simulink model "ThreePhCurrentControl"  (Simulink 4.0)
settings: Solver=ode23  StartTime=-eps  StopTime=0.2  FixedStep=0.000001  RelTol=1e-3
undefined symbols (not defined in the file or in its folder): di, Element, L, R, sfunxy, Symmetrized, Ts, Udc, Upp, Warning
libraries: simulink3 x1

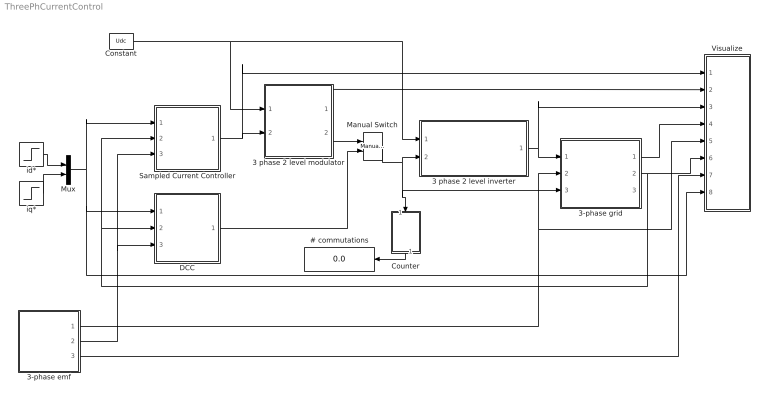
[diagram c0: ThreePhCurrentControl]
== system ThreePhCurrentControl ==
  # commutations : Display
  3 phase 2 level inverter : Subsystem  SimViewingDevice=off
  3 phase 2 level modulator : Subsystem  SimViewingDevice=off  mask{type=Symmetrized, Random=Fixed frequency, Ts=Ts}
      mask prompts: type "Sinus, Symmetrized or Minimum switch modulation"; Random "Fixed or random modulation?"; Ts "Sampling interval"
      mask help: Carrier Wave modulator that uses either fixed frequency modulation or random modulation. The fixed frequency modulation uses 1/(2Ts) as modulation frequency. The random modulation selects the modulatio frequency by random every sampling instant. The selection uses either 1/Ts, 1/(2Ts) or 1/(3Ts) as carrier wave frequency.
  3-phase emf : Subsystem  SimViewingDevice=off  mask{Upp=Upp, freq=50, Tc=0.1e-3}
      mask prompts: Upp "U_phase_to_phase [RMS]"; freq "Frequency"; Tc "Sampling time"
  3-phase grid : Subsystem  SimViewingDevice=off  mask{L=L, R=R}
      mask prompts: L "Inductance [H]"; R "Resistance [ohm]"
  Constant : Constant  Value=Udc
  Counter : Subsystem  Orientation=down  SimViewingDevice=off
  DCC : Subsystem  SimViewingDevice=off
  Manual Switch : simulink3/Nonlinear/Manual Switch  sw=0  action=0
  Mux : Mux  Inputs=2
  Sampled Current Controller : Subsystem  SimViewingDevice=off  mask{R=R, L=L, Kp=(L/Ts+R/2), Ti=L/R+Ts/2, Ts=Ts, Umax=Udc, Umin=-Udc, SlowFast=Slow Computer}
      mask prompts: R "Load resistance"; L "Load inductance"; Kp "Controller gain"; Ti "Integral Time Constant"; Ts "Sampling time [s]"; Umax "Max output signal"; Umin "Min output signal"; SlowFast "Controller type"
  Visualize : Subsystem  SimViewingDevice=off
  id* : Step  Time=0.0105  Before=0  After=-10  SampleTime=0
  iq* : Step  Time=0.0055  Before=0  After=10  SampleTime=0
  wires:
  3 phase 2 level inverter/1(va,b,c) -> 3-phase grid/1(va,b,c), Visualize/3(v)
  Sampled Current Controller/1(u*) -> 3 phase 2 level modulator/2(uabc*), Visualize/1(u*)
  Constant/1 -> 3 phase 2 level inverter/1(Udc), 3 phase 2 level modulator/1(Udc)
  Counter/1(#) -> # commutations/1
  3 phase 2 level modulator/2(sa,b,c) -> Manual Switch/1
  Manual Switch/1 -> 3 phase 2 level inverter/2(sa,b,c), Counter/1(sa,b,c), 3-phase grid/3(s)
  DCC/1(sa,b,c) -> Manual Switch/2
  3 phase 2 level modulator/1(mod) -> Visualize/2(mod)
  3-phase emf/1(e_line) -> 3-phase grid/2(e_line), Visualize/5(e)
  3-phase grid/1(u_ab) -> Visualize/4("u ")
  3-phase grid/2(i_ab) -> Visualize/6(i), DCC/2(Act_ab), Sampled Current Controller/2(Act_ab)
  3-phase emf/3(Theta_line) -> Visualize/7(theta)
  3-phase emf/2(Psi_line) -> DCC/3(psi), Sampled Current Controller/3(psi)
  id*/1 -> Mux/1
  iq*/1 -> Mux/2
  Mux/1 -> Sampled Current Controller/1(Ref_dq), DCC/1(Ref_dq), Visualize/8(i*dq)

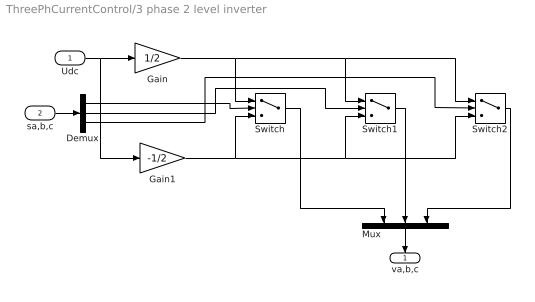
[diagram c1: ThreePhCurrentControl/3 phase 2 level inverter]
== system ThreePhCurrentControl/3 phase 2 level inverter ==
  Udc : Inport  Port=1  PortDimensions=-1  SampleTime=-1  DataType=auto
  sa,b,c : Inport  Port=2  PortDimensions=-1  SampleTime=-1  DataType=auto
  Demux : Demux  Outputs=3  BusSelectionMode=off
  Gain : Gain  Gain=1/2  Multiplication=Element-wise(K.*u)  SaturateOnIntegerOverflow=on
  Gain1 : Gain  Gain=-1/2  Multiplication=Element-wise(K.*u)  SaturateOnIntegerOverflow=on
  Mux : Mux  Orientation=down  Inputs=3
  Switch : Switch  Threshold=0
  Switch1 : Switch  Threshold=0
  Switch2 : Switch  Threshold=0
  va,b,c : Outport  Orientation=down  Port=1  InitialOutput=0
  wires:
  Gain/1 -> Switch/1, Switch1/1, Switch2/1
  Gain1/1 -> Switch/3, Switch1/3, Switch2/3
  Udc/1 -> Gain1/1, Gain/1
  sa,b,c/1 -> Demux/1
  Demux/1 -> Switch/2
  Demux/2 -> Switch1/2
  Demux/3 -> Switch2/2
  Switch/1 -> Mux/1
  Switch1/1 -> Mux/2
  Switch2/1 -> Mux/3
  Mux/1 -> va,b,c/1

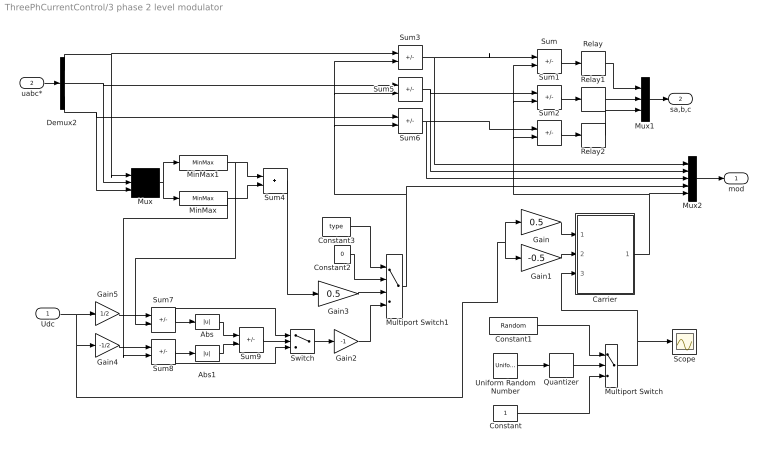
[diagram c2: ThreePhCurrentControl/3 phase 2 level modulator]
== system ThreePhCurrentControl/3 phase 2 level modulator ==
  Udc : Inport  Port=1  PortDimensions=-1  SampleTime=-1  DataType=auto
  uabc* : Inport  Port=2  PortDimensions=-1  SampleTime=-1  DataType=auto
  Abs : Abs  SaturateOnIntegerOverflow=on
  Abs1 : Abs  SaturateOnIntegerOverflow=on
  Carrier : Subsystem  SimViewingDevice=off
  Constant : Constant  Value=1
  Constant1 : Constant  Value=Random
  Constant2 : Constant  Value=0
  Constant3 : Constant  Value=type
  Demux2 : Demux  Outputs=3  BusSelectionMode=off
  Gain : Gain  Gain=0.5  Multiplication=Element-wise(K.*u)  SaturateOnIntegerOverflow=on
  Gain1 : Gain  Gain=-0.5  Multiplication=Element-wise(K.*u)  SaturateOnIntegerOverflow=on
  Gain2 : Gain  Gain=-1  Multiplication=Element-wise(K.*u)  SaturateOnIntegerOverflow=on
  Gain3 : Gain  Gain=0.5  Multiplication=Element-wise(K.*u)  SaturateOnIntegerOverflow=on
  Gain4 : Gain  Gain=-1/2  Multiplication=Element-wise(K.*u)  SaturateOnIntegerOverflow=on
  Gain5 : Gain  Gain=1/2  Multiplication=Element-wise(K.*u)  SaturateOnIntegerOverflow=on
  MinMax : MinMax  Function=min  Inputs=1
  MinMax1 : MinMax  Function=max  Inputs=1
  Multiport Switch : MultiPortSwitch  Inputs=2
  Multiport Switch1 : MultiPortSwitch  Inputs=3
  Mux : Mux  Inputs=3
  Mux1 : Mux  Inputs=3
  Mux2 : Mux  Inputs=5
  Quantizer : Quantizer  QuantizationInterval=1  LinearizeAsGain=on
  Relay : Relay  OnSwitchValue=eps  OffSwitchValue=eps  OnOutputValue=1  OffOutputValue=-1
  Relay1 : Relay  OnSwitchValue=eps  OffSwitchValue=eps  OnOutputValue=1  OffOutputValue=-1
  Relay2 : Relay  OnSwitchValue=eps  OffSwitchValue=eps  OnOutputValue=1  OffOutputValue=-1
  Scope : Scope
  Sum{,1..3,5..8} (8 alike) : Sum  Inputs=+-  SaturateOnIntegerOverflow=on
  Sum4 : Sum  Inputs=++  SaturateOnIntegerOverflow=on
  Sum9 : Sum  Inputs=-+  SaturateOnIntegerOverflow=on
  Switch : Switch  Threshold=0
  Uniform Random Number : UniformRandomNumber  Minimum=1  Maximum=3  Seed=0.9874  SampleTime=Ts
  mod : Outport  Port=1  InitialOutput=0
  sa,b,c : Outport  Port=2  InitialOutput=0
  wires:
  Carrier/1(um) -> Sum2/2, Sum1/2, Sum/2, Mux2/5
  Gain1/1 -> Carrier/2(Umin)
  Gain/1 -> Carrier/1(Umax)
  Sum/1 -> Relay/1
  Relay1/1 -> Mux1/2
  Sum1/1 -> Relay1/1
  Relay2/1 -> Mux1/3
  Sum2/1 -> Relay2/1
  Quantizer/1 -> Multiport Switch/2
  Uniform Random Number/1 -> Quantizer/1
  Constant/1 -> Multiport Switch/3
  Multiport Switch/1 -> Carrier/3(x), Scope/1
  Constant1/1 -> Multiport Switch/1
  Sum3/1 -> Mux2/1, Sum/1
  Sum5/1 -> Mux2/2, Sum1/1
  Sum6/1 -> Mux2/3, Sum2/1
  Demux2/1 -> Sum3/1, Mux/1
  Demux2/2 -> Sum5/1, Mux/2
  Demux2/3 -> Sum6/1, Mux/3
  Mux/1 -> MinMax1/1, MinMax/1
  MinMax1/1 -> Sum4/1, Sum7/2
  MinMax/1 -> Sum4/2, Sum8/2
  Udc/1 -> Gain5/1, Gain4/1, Gain1/1, Gain/1
  Gain4/1 -> Sum8/1
  Sum7/1 -> Abs/1, Switch/1
  Sum8/1 -> Abs1/1, Switch/3
  Abs/1 -> Sum9/1
  Abs1/1 -> Sum9/2
  Sum9/1 -> Switch/2
  Sum4/1 -> Gain3/1
  Switch/1 -> Gain2/1
  Constant3/1 -> Multiport Switch1/1
  Constant2/1 -> Multiport Switch1/2
  Gain3/1 -> Multiport Switch1/3
  Gain2/1 -> Multiport Switch1/4
  Multiport Switch1/1 -> Sum5/2, Sum3/2, Sum6/2, Mux2/4
  Gain5/1 -> Sum7/1
  uabc*/1 -> Demux2/1
  Relay/1 -> Mux1/1
  Mux1/1 -> sa,b,c/1
  Mux2/1 -> mod/1

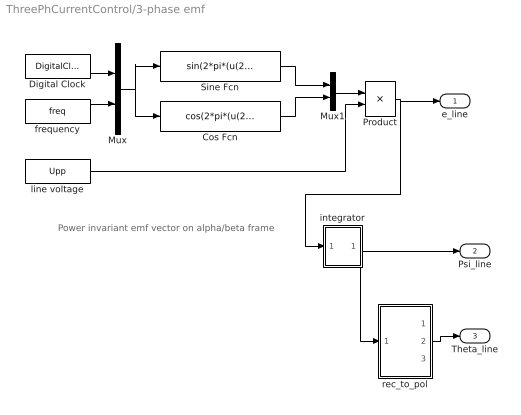
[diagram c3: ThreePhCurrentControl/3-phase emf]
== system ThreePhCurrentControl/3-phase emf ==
  note: Power invariant emf vector on alpha/beta frame
  Cos Fcn : Fcn  Expr=cos(2*pi*(u(2))*u(1))
  Digital Clock : DigitalClock  SampleTime=Tc
  Mux : Mux  Inputs=2
  Mux1 : Mux  Inputs=2
  Product : Product  Inputs=2  Multiplication=Element-wise(.*)  SaturateOnIntegerOverflow=on
  Sine Fcn : Fcn  Expr=sin(2*pi*(u(2))*u(1)-pi)
  frequency : Constant  Value=freq
  integrator : Subsystem  SimViewingDevice=off
  line voltage : Constant  Value=Upp
  rec_to_pol : Subsystem  SimViewingDevice=off
  e_line : Outport  Port=1  InitialOutput=0
  Psi_line : Outport  Port=2  InitialOutput=0
  Theta_line : Outport  Port=3  InitialOutput=0
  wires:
  Product/1 -> e_line/1, integrator/1(In1)
  Mux1/1 -> Product/1
  Cos Fcn/1 -> Mux1/2
  Sine Fcn/1 -> Mux1/1
  Mux/1 -> Cos Fcn/1, Sine Fcn/1
  Digital Clock/1 -> Mux/1
  frequency/1 -> Mux/2
  line voltage/1 -> Product/2
  integrator/1(Out1) -> Psi_line/1, rec_to_pol/1(rect)
  rec_to_pol/2(angle) -> Theta_line/1

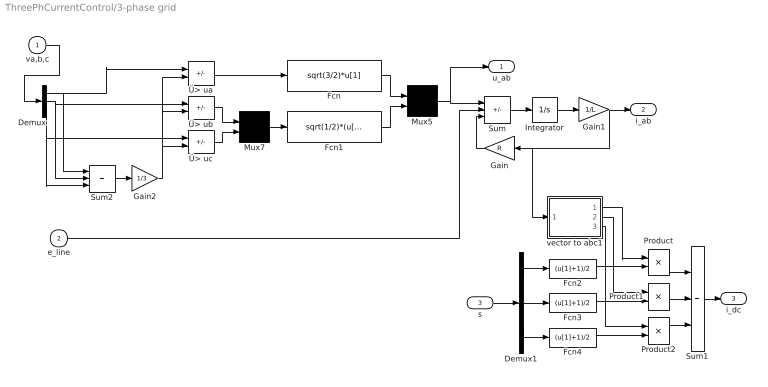
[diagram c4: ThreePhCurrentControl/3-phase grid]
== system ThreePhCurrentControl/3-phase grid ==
  va,b,c : Inport  Port=1  PortDimensions=-1  SampleTime=-1  DataType=auto
  e_line : Inport  Port=2  PortDimensions=-1  SampleTime=-1  DataType=auto
  s : Inport  Port=3  PortDimensions=-1  SampleTime=-1  DataType=auto
  Demux : Demux  Outputs=3  BusSelectionMode=off
  Demux1 : Demux  Outputs=3  BusSelectionMode=off
  Fcn : Fcn  Expr=sqrt(3/2)*u[1]
  Fcn1 : Fcn  Expr=sqrt(1/2)*(u[1]-u[2])
  Fcn2 : Fcn  Expr=(u[1]+1)/2
  Fcn3 : Fcn  Expr=(u[1]+1)/2
  Fcn4 : Fcn  Expr=(u[1]+1)/2
  Gain : Gain  Orientation=left  Gain=R  Multiplication=Element-wise(K.*u)  SaturateOnIntegerOverflow=on
  Gain1 : Gain  Gain=1/L  Multiplication=Element-wise(K.*u)  SaturateOnIntegerOverflow=on
  Gain2 : Gain  Gain=1/3  Multiplication=Element-wise(K.*u)  SaturateOnIntegerOverflow=on
  Integrator : Integrator  ExternalReset=none  InitialConditionSource=internal  InitialCondition=0  LimitOutput=off  UpperSaturationLimit=inf  LowerSaturationLimit=-inf  ShowSaturationPort=off  ShowStatePort=off  AbsoluteTolerance=auto
  Mux5 : Mux  Inputs=2
  Mux7 : Mux  Inputs=2
  Product : Product  Inputs=2  Multiplication=Element-wise(.*)  SaturateOnIntegerOverflow=on
  Product1 : Product  Inputs=2  Multiplication=Element-wise(.*)  SaturateOnIntegerOverflow=on
  Product2 : Product  Inputs=2  Multiplication=Element-wise(.*)  SaturateOnIntegerOverflow=on
  Sum : Sum  Inputs=+--  SaturateOnIntegerOverflow=on
  Sum1 : Sum  Inputs=+++  SaturateOnIntegerOverflow=on
  Sum2 : Sum  Inputs=+++  SaturateOnIntegerOverflow=on
  vector to abc1 : Subsystem  SimViewingDevice=off
  Ü> ua : Sum  Inputs=+-  SaturateOnIntegerOverflow=on
  Ü> ub : Sum  Inputs=+-  SaturateOnIntegerOverflow=on
  Ü> uc : Sum  Inputs=+-  SaturateOnIntegerOverflow=on
  u_ab : Outport  Port=1  InitialOutput=0
  i_ab : Outport  Port=2  InitialOutput=0
  i_dc : Outport  Port=3
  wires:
  Gain1/1 -> i_ab/1, Gain/1, vector to abc1/1(vect)
  Integrator/1 -> Gain1/1
  Gain/1 -> Sum/3
  Sum/1 -> Integrator/1
  Fcn1/1 -> Mux5/2
  Fcn/1 -> Mux5/1
  Mux5/1 -> Sum/1, u_ab/1
  Mux7/1 -> Fcn1/1
  Ü> uc/1 -> Mux7/2
  Ü> ub/1 -> Mux7/1
  Ü> ua/1 -> Fcn/1
  Gain2/1 -> Ü> uc/2, Ü> ub/2, Ü> ua/2
  Demux/2 -> Ü> ub/1, Sum2/2
  Sum2/1 -> Gain2/1
  Demux/3 -> Ü> uc/1, Sum2/3
  Demux/1 -> Ü> ua/1, Sum2/1
  va,b,c/1 -> Demux/1
  Demux1/2 -> Fcn3/1
  Demux1/1 -> Fcn2/1
  Demux1/3 -> Fcn4/1
  s/1 -> Demux1/1
  Sum1/1 -> i_dc/1
  Product2/1 -> Sum1/3
  Product1/1 -> Sum1/2
  Product/1 -> Sum1/1
  vector to abc1/1(a) -> Product/1
  vector to abc1/2(b) -> Product1/1
  vector to abc1/3(c) -> Product2/1
  Fcn4/1 -> Product2/2
  Fcn3/1 -> Product1/2
  Fcn2/1 -> Product/2
  e_line/1 -> Sum/2

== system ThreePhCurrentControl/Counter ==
  sa,b,c : Inport  Port=1  PortDimensions=-1  SampleTime=-1  DataType=auto
  Demux : Demux  Outputs=3  BusSelectionMode=off
  Subsystem : Subsystem  TreatAsAtomicUnit=on  SimViewingDevice=off
  Subsystem1 : Subsystem  TreatAsAtomicUnit=on  SimViewingDevice=off
  Subsystem2 : Subsystem  TreatAsAtomicUnit=on  SimViewingDevice=off
  Sum : Sum  Inputs=+++  SaturateOnIntegerOverflow=on
  # : Outport  Port=1
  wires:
  Sum/1 -> #/1
  Subsystem/1(Out1) -> Sum/2
  Subsystem2/1(Out1) -> Sum/1
  Subsystem1/1(Out1) -> Sum/3
  sa,b,c/1 -> Demux/1
  Demux/2 -> Subsystem/Trigger
  Demux/3 -> Subsystem1/Trigger
  Demux/1 -> Subsystem2/Trigger

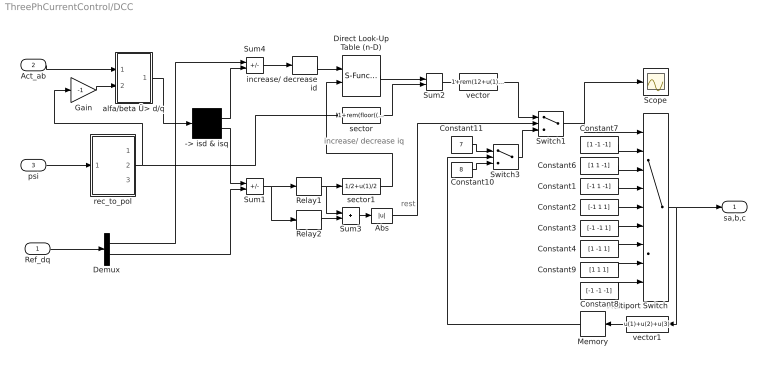
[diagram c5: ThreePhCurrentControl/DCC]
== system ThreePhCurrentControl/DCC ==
  note: increase/ decrease iq
  note: rest
  Ref_dq : Inport  Port=1  PortDimensions=-1  SampleTime=-1  DataType=auto
  Act_ab : Inport  Port=2  PortDimensions=-1  SampleTime=-1  DataType=auto
  psi : Inport  Port=3  PortDimensions=-1  SampleTime=-1  DataType=auto
  -> isd & isq : Demux  Outputs=2  BusSelectionMode=off
  Abs : Abs  SaturateOnIntegerOverflow=on
  Constant1 : Constant  Value=[-1 1 -1]
  Constant10 : Constant  Value=8
  Constant11 : Constant  Value=7
  Constant2 : Constant  Value=[-1 1 1]
  Constant3 : Constant  Value=[-1 -1 1]
  Constant4 : Constant  Value=[1 -1 1]
  Constant6 : Constant  Value=[1 1 -1]
  Constant7 : Constant  Value=[1 -1 -1]
  Constant8 : Constant  Value=[-1 -1 -1]
  Constant9 : Constant  Value=[1 1 1]
  Demux : Demux  Outputs=2  BusSelectionMode=off
  Direct Look-Up Table (n-D) : S-Function  FunctionName=sfun_nddirectlook  Parameters=numInputs,mxTable,clipFlag,tabIsInput,numTDims  PortCounts=[]  SFunctionModules=''  mask(LookupNDDirect){maskTabDims=2, explicitNumDims=1, outDims=Element, tabIsInput=off, mxTable=[4 2;5 1], clipFlag=Warning}
      mask prompts: maskTabDims "Number of table dimensions:"; explicitNumDims "Explicit number of table dimensions:"; outDims "Inputs select this object from table:"; tabIsInput "Make table an input"; mxTable "Table data:"; clipFlag "Action for out of range input:"
      mask help: Table member selection. Inputs are zero-based indices into the table, e.g., an input of 3 returns the fourth element in that dimension. Block can also be used to select a column or 2-D matrix out of the table.
      mask init:
      | if tabIsInput == 1
      |   tWhat = ' T';
      |   yT = 1/(3+maskTabDims-outDims);
      | else
      |   tWhat = ' ';
      |   yT = 0;
      | end
      | if maskTabDims >= 5
      |   numTDims = explicitNumDims;
      | else
      |   numTDims = maskTabDims;
      | end
      | numInputs =  numTDims - (outDims-1);
      | if strcmp(get_param(bdroot(gcb),'BlockDiagramType'),'library')
      |   dimsChar = 'n';
      | else
      |   dimsChar = sprintf('%d',numTDims);
      | end
      | [x,y] = nddirectico('plotdata', numTDims, tabIsInput, outDims);
      | xp = x((end-3):end); yp = y((end-3):end);
      | x = x(1:(end-4)); y = y(1:(end-4));
  Gain : Gain  Gain=-1  Multiplication=Element-wise(K.*u)  SaturateOnIntegerOverflow=on
  Memory : Memory  Orientation=left  X0=0  InheritSampleTime=off
  Multiport Switch : MultiPortSwitch  Inputs=8
  Relay1 : Relay  OnSwitchValue=di/2  OffSwitchValue=-di/2  OnOutputValue=1  OffOutputValue=-1
  Relay2 : Relay  OnSwitchValue=1.3*di/2  OffSwitchValue=-1.3*di/2  OnOutputValue=1  OffOutputValue=-1
  Scope : Scope
  Sum1 : Sum  Inputs=-+  SaturateOnIntegerOverflow=on
  Sum2 : Sum  Inputs=++  SaturateOnIntegerOverflow=on
  Sum3 : Sum  Inputs=++  SaturateOnIntegerOverflow=on
  Sum4 : Sum  Inputs=+-  SaturateOnIntegerOverflow=on
  Switch1 : Switch  Threshold=1
  Switch3 : Switch  Threshold=1
  alfa/beta Ü> d/q : Subsystem  SimViewingDevice=off
  increase/ decrease id : Relay  OnSwitchValue=di/2  OffSwitchValue=-di/2  OnOutputValue=1  OffOutputValue=0
  rec_to_pol : Subsystem  SimViewingDevice=off
  sector : Fcn  Expr=1+rem(floor((2*pi+u(1)+pi/6)/(pi/3+eps)),6)
  sector1 : Fcn  Expr=1/2+u(1)/2
  vector : Fcn  Expr=1+rem(12+u(1)-1,6)
  vector1 : Fcn  Orientation=left  Expr=u(1)+u(2)+u(3)
  sa,b,c : Outport  Port=1
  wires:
  Gain/1 -> alfa/beta Ü> d/q/2(angle)
  Act_ab/1 -> alfa/beta Ü> d/q/1(vect)
  alfa/beta Ü> d/q/1(Out) -> -> isd & isq/1
  psi/1 -> rec_to_pol/1(rect)
  -> isd & isq/1 -> Sum4/2
  rec_to_pol/2(angle) -> Gain/1, sector/1
  Multiport Switch/1 -> vector1/1, sa,b,c/1
  Switch1/1 -> Multiport Switch/1, Scope/1
  vector/1 -> Switch1/1
  Sum4/1 -> increase/ decrease id/1
  Sum2/1 -> vector/1
  vector1/1 -> Memory/1
  -> isd & isq/2 -> Sum1/1
  Constant10/1 -> Switch3/3
  Constant11/1 -> Switch3/1
  Memory/1 -> Switch3/2
  Switch3/1 -> Switch1/3
  Relay1/1 -> Sum3/1, sector1/1
  Relay2/1 -> Sum3/2
  Sum3/1 -> Abs/1
  Sum1/1 -> Relay1/1, Relay2/1
  Abs/1 -> Switch1/2
  increase/ decrease id/1 -> Direct Look-Up Table (n-D)/1
  sector1/1 -> Direct Look-Up Table (n-D)/2
  sector/1 -> Sum2/2
  Direct Look-Up Table (n-D)/1 -> Sum2/1
  Constant6/1 -> Multiport Switch/3
  Constant7/1 -> Multiport Switch/2
  Constant8/1 -> Multiport Switch/9
  Constant9/1 -> Multiport Switch/8
  Constant1/1 -> Multiport Switch/4
  Constant2/1 -> Multiport Switch/5
  Constant3/1 -> Multiport Switch/6
  Constant4/1 -> Multiport Switch/7
  Ref_dq/1 -> Demux/1
  Demux/1 -> Sum4/1
  Demux/2 -> Sum1/2

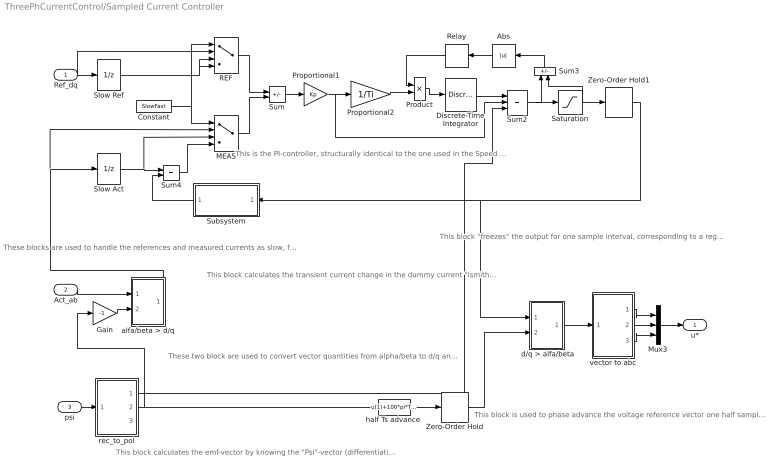
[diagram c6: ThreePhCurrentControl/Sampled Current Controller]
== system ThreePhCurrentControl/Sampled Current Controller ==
  note: These blocks are used to handle the references and measured currents as slow, fast or fast computer with Smith predictor.
  note: This block calculates the transient current change in the dummy current "ismith" The smith predictor calculates the current change that would have been measured if the computer was "fast", i.e. without the delay that a slow computer has. The calculated current change equals the real current change, but informing the controller one sampling interval earlier, thus allowing a high (deadbeat) gain.
  note: This is the PI-controller, structurally identical to the one used in the Speed Controller
  note: This block "freezes" the output for one sample interval, corresponding to a register in a microcontroller where the reference voltages are written once every sampling inteval.
  note: These two block are used to convert vector quantities from alpha/beta to d/q and back again. Note that they are identical, but use the angle with opposite sign.
  note: This block calculates the emf-vector by knowing the "Psi"-vector (differentiation) and calculates the emf- components in the d/q-plane (ideally there is only "eq" whilse "ed"=0). It alse calculates the angle of the "Psi"- vector, used to orient the d/q-plane.
  note: This block is used to phase advance the voltage reference vector one half sample period. It is done to compensate for the fact that the "reality" is turning during the same sample period as the voltage references are being held constant. In the beginning of the sample period, the voltage reference will be 1/2 sample period ahead of reality, and in the end of the sample period it will be 1/2 period behind. In average, it will be in the correct position relative to reality.
  Ref_dq : Inport  Port=1  PortDimensions=-1  SampleTime=-1  DataType=auto
  Act_ab : Inport  Port=2  PortDimensions=-1  SampleTime=-1  DataType=auto
  psi : Inport  Port=3  PortDimensions=-1  SampleTime=-1  DataType=auto
  " d/q > alfa/beta" : Subsystem  SimViewingDevice=off
  Abs : Abs  Orientation=left  SaturateOnIntegerOverflow=on
  Constant : Constant  Value=SlowFast
  Discrete-Time Integrator : DiscreteIntegrator  IntegratorMethod=Forward Euler  ExternalReset=none  InitialConditionSource=internal  InitialCondition=0  LimitOutput=on  UpperSaturationLimit=Umax  LowerSaturationLimit=Umin  ShowSaturationPort=off  ShowStatePort=off  SampleTime=Ts
  Gain : Gain  Gain=-1  Multiplication=Element-wise(K.*u)  SaturateOnIntegerOverflow=on
  MEAS : MultiPortSwitch  Inputs=3
  Mux3 : Mux  Inputs=3
  Product : Product  Inputs=2  Multiplication=Element-wise(.*)  SaturateOnIntegerOverflow=on
  Proportional1 : Gain  Gain=Kp  Multiplication=Element-wise(K.*u)  SaturateOnIntegerOverflow=on
  Proportional2 : Gain  Gain=1/Ti  Multiplication=Element-wise(K.*u)  SaturateOnIntegerOverflow=on
  REF : MultiPortSwitch  Inputs=3
  Relay : Relay  Orientation=left  OnSwitchValue=eps  OffSwitchValue=eps  OnOutputValue=0  OffOutputValue=1
  Saturation : Saturate  UpperLimit=Umax  LowerLimit=Umin  LinearizeAsGain=on
  Slow Act : UnitDelay  X0=0  SampleTime=Ts
  Slow Ref : UnitDelay  X0=0  SampleTime=Ts
  Subsystem : Subsystem  Orientation=left  SimViewingDevice=off
  Sum : Sum  Inputs=+-  SaturateOnIntegerOverflow=on
  Sum2 : Sum  Inputs=+++  SaturateOnIntegerOverflow=on
  Sum3 : Sum  Orientation=up  Inputs=+-  SaturateOnIntegerOverflow=on
  Sum4 : Sum  Inputs=++  SaturateOnIntegerOverflow=on
  Zero-Order Hold : ZeroOrderHold  SampleTime=Ts
  Zero-Order Hold1 : ZeroOrderHold  SampleTime=Ts
  alfa/beta > d/q : Subsystem  SimViewingDevice=off
  "half Ts advance " : Fcn  Expr=u(1)+100*pi*Ts/2
  rec_to_pol : Subsystem  SimViewingDevice=off
  vector to abc : Subsystem  SimViewingDevice=off
  u* : Outport  Port=1
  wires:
  Discrete-Time Integrator/1 -> Sum2/1
  Proportional1/1 -> Proportional2/1, Sum2/2
  Sum/1 -> Proportional1/1
  Sum2/1 -> Saturation/1, Sum3/1
  Saturation/1 -> Zero-Order Hold1/1, Sum3/2
  Proportional2/1 -> Product/2
  Product/1 -> Discrete-Time Integrator/1
  Relay/1 -> Product/1
  Ref_dq/1 -> REF/2, Slow Ref/1
  Zero-Order Hold1/1 -> Subsystem/1(u), " d/q > alfa/beta"/1(vect)
  Slow Act/1 -> Sum4/1, MEAS/3
  Subsystem/1(di_smith) -> Sum4/2
  Constant/1 -> MEAS/1, REF/1
  Slow Ref/1 -> REF/3, REF/4
  REF/1 -> Sum/1
  Sum4/1 -> MEAS/4
  MEAS/1 -> Sum/2
  Sum3/1 -> Abs/1
  Abs/1 -> Relay/1
  Gain/1 -> alfa/beta > d/q/2(angle)
  Act_ab/1 -> alfa/beta > d/q/1(vect)
  psi/1 -> rec_to_pol/1(rect)
  rec_to_pol/2(angle) -> Gain/1, "half Ts advance "/1
  "half Ts advance "/1 -> Zero-Order Hold/1
  Zero-Order Hold/1 -> " d/q > alfa/beta"/2(angle)
  " d/q > alfa/beta"/1(Out) -> vector to abc/1(vect)
  vector to abc/1(a) -> Mux3/1
  vector to abc/2(b) -> Mux3/2
  vector to abc/3(c) -> Mux3/3
  alfa/beta > d/q/1(Out) -> Slow Act/1, MEAS/2
  Mux3/1 -> u*/1
  rec_to_pol/1(e) -> Sum2/3

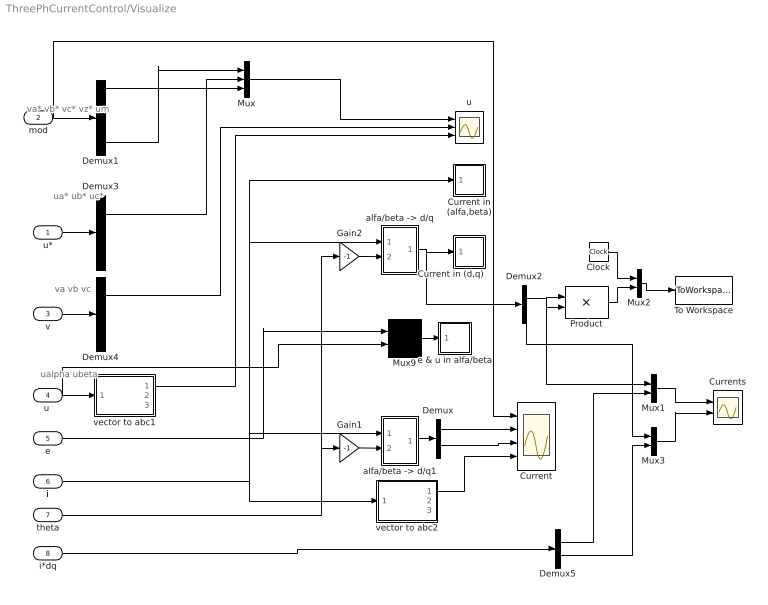
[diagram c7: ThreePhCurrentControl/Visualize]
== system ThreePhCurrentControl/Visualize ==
  note: va* vb* vc* vz* um
  note: ua* ub* uc*
  note: ualpha ubeta
  note: va vb vc
  u* : Inport  Port=1  PortDimensions=-1  SampleTime=-1  DataType=auto
  mod : Inport  Port=2  PortDimensions=-1  SampleTime=-1  DataType=auto
  v : Inport  Port=3  PortDimensions=-1  SampleTime=-1  DataType=auto
  "u " : Inport  Port=4  PortDimensions=-1  SampleTime=-1  DataType=auto
  e : Inport  Port=5  PortDimensions=-1  SampleTime=-1  DataType=auto
  i : Inport  Port=6  PortDimensions=-1  SampleTime=-1  DataType=auto
  theta : Inport  Port=7  PortDimensions=-1  SampleTime=-1  DataType=auto
  i*dq : Inport  Port=8  PortDimensions=-1  SampleTime=-1  DataType=auto
  Clock : Clock
  Current : Scope  NumInputPorts=4
  Current in (alfa,beta) : Subsystem  LoadFcn=sfunxy([],[],[],'LoadBlock')  StartFcn=sfunxy([],[],[],'Start')  StopFcn=sfunxy([],[],[],'Stop')  SimViewingDevice=off  mask(XY scope.){xmin=-20, xmax=20, ymin=-20, ymax=20, st=-1}
      mask prompts: xmin "x-min:"; xmax "x-max:"; ymin "y-min:"; ymax "y-max:"; st "Sample time:"
      mask help: XY scope using MATLAB graph window. First input is used as time base. Enter plotting ranges.
  Current in (d,q) : Subsystem  LoadFcn=sfunxy([],[],[],'LoadBlock')  StartFcn=sfunxy([],[],[],'Start')  StopFcn=sfunxy([],[],[],'Stop')  SimViewingDevice=off  mask(XY scope.){xmin=-20, xmax=20, ymin=-20, ymax=20, st=-1}
      mask prompts: xmin "x-min:"; xmax "x-max:"; ymin "y-min:"; ymax "y-max:"; st "Sample time:"
      mask help: XY scope using MATLAB graph window. First input is used as time base. Enter plotting ranges.
  Currents : Scope  NumInputPorts=2
  Demux : Demux  Outputs=2  BusSelectionMode=off
  Demux1 : Demux  Outputs=5  BusSelectionMode=off
  Demux2 : Demux  Outputs=2  BusSelectionMode=off
  Demux3 : Demux  Outputs=3  BusSelectionMode=off
  Demux4 : Demux  Outputs=3  BusSelectionMode=off
  Demux5 : Demux  Outputs=2  BusSelectionMode=off
  Gain1 : Gain  Gain=-1  Multiplication=Element-wise(K.*u)  SaturateOnIntegerOverflow=on
  Gain2 : Gain  Gain=-1  Multiplication=Element-wise(K.*u)  SaturateOnIntegerOverflow=on
  Mux : Mux  Inputs=3
  Mux{1..3,9} (4 alike) : Mux  Inputs=2
  Product : Product  Inputs=2  Multiplication=Element-wise(.*)  SaturateOnIntegerOverflow=on
  To Workspace : ToWorkspace  VariableName=f1  SampleTime=-1  SaveFormat=Array
  "alfa/beta -> d/q" : Subsystem  SimViewingDevice=off
  "alfa/beta -> d/q1" : Subsystem  SimViewingDevice=off
  e & u in alfa/beta : Subsystem  LoadFcn=sfunxy([],[],[],'LoadBlock')  StartFcn=sfunxy([],[],[],'Start')  StopFcn=sfunxy([],[],[],'Stop')  SimViewingDevice=off  mask(XY scope.){xmin=-300, xmax=300, ymin=-300, ymax=300, st=-1}
      mask prompts: xmin "x-min:"; xmax "x-max:"; ymin "y-min:"; ymax "y-max:"; st "Sample time:"
      mask help: XY scope using MATLAB graph window. First input is used as time base. Enter plotting ranges.
  u : Scope  NumInputPorts=3
  vector to abc1 : Subsystem  SimViewingDevice=off
  vector to abc2 : Subsystem  SimViewingDevice=off
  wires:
  Gain2/1 -> "alfa/beta -> d/q"/2(angle)
  Gain1/1 -> "alfa/beta -> d/q1"/2(angle)
  "alfa/beta -> d/q1"/1(Out) -> Demux/1
  Demux/1 -> Current/2
  Demux/2 -> Current/3
  vector to abc2/1(a) -> Current/4
  mod/1 -> Demux1/1, Current/1
  "alfa/beta -> d/q"/1(Out) -> Current in (d,q)/1(xy), Demux2/1
  Demux1/5 -> Mux/1
  Demux1/1 -> Mux/3
  Mux/1 -> u/1
  u*/1 -> Demux3/1
  "u "/1 -> vector to abc1/1(vect), Mux9/2
  Demux3/1 -> Mux/2
  v/1 -> Demux4/1
  Demux4/1 -> u/2
  vector to abc1/1(a) -> u/3
  i/1 -> Current in (alfa,beta)/1(xy), "alfa/beta -> d/q"/1(vect), "alfa/beta -> d/q1"/1(vect), vector to abc2/1(vect)
  Mux9/1 -> e & u in alfa/beta/1(xy)
  e/1 -> Mux9/1
  theta/1 -> Gain1/1, Gain2/1
  Clock/1 -> Mux2/1
  Product/1 -> Mux2/2
  Mux2/1 -> To Workspace/1
  Demux2/1 -> Product/1, Product/2, Mux1/1
  i*dq/1 -> Demux5/1
  Demux5/1 -> Mux1/2
  Demux2/2 -> Mux3/1
  Demux5/2 -> Mux3/2
  Mux3/1 -> Currents/2
  Mux1/1 -> Currents/1

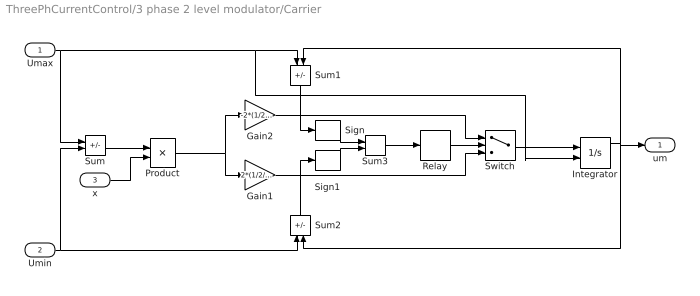
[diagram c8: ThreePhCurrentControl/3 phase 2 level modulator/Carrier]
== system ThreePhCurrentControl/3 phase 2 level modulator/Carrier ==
  Umax : Inport  Port=1  PortDimensions=-1  SampleTime=-1  DataType=auto
  Umin : Inport  Port=2  PortDimensions=-1  SampleTime=-1  DataType=auto
  x : Inport  Port=3  PortDimensions=-1  SampleTime=-1  DataType=auto
  Gain1 : Gain  Gain=2*(1/2/Ts)  Multiplication=Element-wise(K.*u)  SaturateOnIntegerOverflow=on
  Gain2 : Gain  Gain=-2*(1/2/Ts)  Multiplication=Element-wise(K.*u)  SaturateOnIntegerOverflow=on
  Integrator : Integrator  ExternalReset=none  InitialConditionSource=external  InitialCondition=0  LimitOutput=off  UpperSaturationLimit=inf  LowerSaturationLimit=-inf  ShowSaturationPort=off  ShowStatePort=off  AbsoluteTolerance=auto
  Product : Product  Inputs=2  Multiplication=Element-wise(.*)  SaturateOnIntegerOverflow=on
  Relay : Relay  OnSwitchValue=1  OffSwitchValue=-1  OnOutputValue=1  OffOutputValue=-1
  Sign : Signum
  Sign1 : Signum
  Sum : Sum  Inputs=+-  SaturateOnIntegerOverflow=on
  Sum1 : Sum  Orientation=down  Inputs=-+  SaturateOnIntegerOverflow=on
  Sum2 : Sum  Orientation=up  Inputs=-+  SaturateOnIntegerOverflow=on
  Sum3 : Sum  Inputs=++  SaturateOnIntegerOverflow=on
  Switch : Switch  Threshold=0
  um : Outport  Port=1
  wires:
  Switch/1 -> Integrator/1
  Umax/1 -> Sum/1, Sum1/1, Integrator/2
  Umin/1 -> Sum/2, Sum2/1
  Gain2/1 -> Switch/1
  Gain1/1 -> Switch/3
  Integrator/1 -> Sum1/2, um/1, Sum2/2
  Sum1/1 -> Sign/1
  Sum2/1 -> Sign1/1
  Sign/1 -> Sum3/1
  Sign1/1 -> Sum3/2
  Sum3/1 -> Relay/1
  Relay/1 -> Switch/2
  Sum/1 -> Product/1
  Product/1 -> Gain2/1, Gain1/1
  x/1 -> Product/2

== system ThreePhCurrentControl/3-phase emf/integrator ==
  note: Power invariant emf vector on alpha/beta frame
  In1 : Inport  Port=1  PortDimensions=-1  SampleTime=-1  DataType=auto
  Demux : Demux  Outputs=2  BusSelectionMode=off
  Integrator1 : Integrator  ExternalReset=none  InitialConditionSource=internal  InitialCondition=Upp/(2*pi*freq)  LimitOutput=off  UpperSaturationLimit=inf  LowerSaturationLimit=-inf  ShowSaturationPort=off  ShowStatePort=off  AbsoluteTolerance=auto
  Integrator2 : Integrator  ExternalReset=none  InitialConditionSource=internal  InitialCondition=0  LimitOutput=off  UpperSaturationLimit=inf  LowerSaturationLimit=-inf  ShowSaturationPort=off  ShowStatePort=off  AbsoluteTolerance=auto
  Mux : Mux  Inputs=2
  Out1 : Outport  Port=1
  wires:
  In1/1 -> Demux/1
  Mux/1 -> Out1/1
  Integrator2/1 -> Mux/2
  Integrator1/1 -> Mux/1
  Demux/2 -> Integrator2/1
  Demux/1 -> Integrator1/1

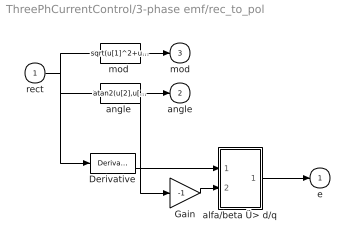
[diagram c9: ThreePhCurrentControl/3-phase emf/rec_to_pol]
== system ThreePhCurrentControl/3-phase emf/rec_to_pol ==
  rect : Inport  Port=1  PortDimensions=-1  SampleTime=-1  DataType=auto
  Derivative : Derivative
  Gain : Gain  Gain=-1  Multiplication=Element-wise(K.*u)  SaturateOnIntegerOverflow=on
  alfa/beta Ü> d/q : Subsystem  SimViewingDevice=off
  "angle " : Fcn  Expr=atan2(u[2],u[1])
  "mod " : Fcn  Expr=sqrt(u[1]^2+u[2]^2)
  e : Outport  Port=1  InitialOutput=0
  angle : Outport  Port=2  InitialOutput=0
  mod : Outport  Port=3  InitialOutput=0
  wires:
  "angle "/1 -> angle/1, Gain/1
  rect/1 -> "angle "/1, "mod "/1, Derivative/1
  "mod "/1 -> mod/1
  Gain/1 -> alfa/beta Ü> d/q/2(angle)
  Derivative/1 -> alfa/beta Ü> d/q/1(vect)
  alfa/beta Ü> d/q/1(Out) -> e/1

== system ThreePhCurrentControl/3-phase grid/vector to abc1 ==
  vect : Inport  Port=1  PortDimensions=-1  SampleTime=-1  DataType=auto
  Ü> a : Fcn  Expr=sqrt(2/3)*u[1]
  Ü> b : Fcn  Expr=-sqrt(1/6)*u[1]+sqrt(1/2)*u[2]
  Ü> c : Fcn  Expr=-sqrt(1/6)*u[1]-sqrt(1/2)*u[2]
  a : Outport  Port=1  InitialOutput=0
  b : Outport  Port=2  InitialOutput=0
  c : Outport  Port=3  InitialOutput=0
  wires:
  vect/1 -> Ü> b/1, Ü> a/1, Ü> c/1
  Ü> b/1 -> b/1
  Ü> c/1 -> c/1
  Ü> a/1 -> a/1

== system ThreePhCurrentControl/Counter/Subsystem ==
  Trigger : TriggerPort  TriggerType=either  OutputDataType=auto
  Constant : Constant  Value=1
  Memory : Memory  Orientation=left  X0=0  InheritSampleTime=on
  Sum : Sum  Inputs=++  SaturateOnIntegerOverflow=on
  Out1 : Outport  Port=1
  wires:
  Sum/1 -> Memory/1, Out1/1
  Memory/1 -> Sum/2
  Constant/1 -> Sum/1

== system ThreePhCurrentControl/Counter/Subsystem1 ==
  Trigger : TriggerPort  TriggerType=either  OutputDataType=auto
  Constant : Constant  Value=1
  Memory : Memory  Orientation=left  X0=0  InheritSampleTime=on
  Sum : Sum  Inputs=++  SaturateOnIntegerOverflow=on
  Out1 : Outport  Port=1
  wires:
  Constant/1 -> Sum/1
  Memory/1 -> Sum/2
  Sum/1 -> Memory/1, Out1/1

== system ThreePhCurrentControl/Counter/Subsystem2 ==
  Trigger : TriggerPort  TriggerType=either  OutputDataType=auto
  Constant : Constant  Value=1
  Memory : Memory  Orientation=left  X0=0  InheritSampleTime=on
  Sum : Sum  Inputs=++  SaturateOnIntegerOverflow=on
  Out1 : Outport  Port=1
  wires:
  Sum/1 -> Memory/1, Out1/1
  Memory/1 -> Sum/2
  Constant/1 -> Sum/1

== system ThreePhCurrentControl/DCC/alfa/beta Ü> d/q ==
  vect : Inport  Port=1  PortDimensions=-1  SampleTime=-1  DataType=auto
  angle : Inport  Port=2  PortDimensions=-1  SampleTime=-1  DataType=auto
  Fcn : Fcn  Expr=u[1]*cos(u[3])-u[2]*sin(u[3])
  Fcn1 : Fcn  Expr=u[1]*sin(u[3])+u[2]*cos(u[3])
  Mux : Mux  Inputs=2
  Mux1 : Mux  Inputs=2
  Out : Outport  Port=1  InitialOutput=0
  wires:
  vect/1 -> Mux/1
  angle/1 -> Mux/2
  Mux/1 -> Fcn/1, Fcn1/1
  Fcn/1 -> Mux1/1
  Fcn1/1 -> Mux1/2
  Mux1/1 -> Out/1

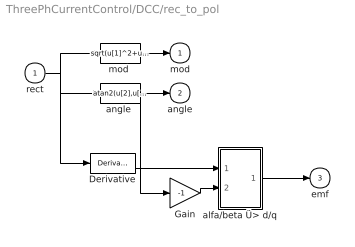
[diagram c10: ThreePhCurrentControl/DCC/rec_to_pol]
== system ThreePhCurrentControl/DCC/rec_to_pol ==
  rect : Inport  Port=1  PortDimensions=-1  SampleTime=-1  DataType=auto
  Derivative : Derivative
  Gain : Gain  Gain=-1  Multiplication=Element-wise(K.*u)  SaturateOnIntegerOverflow=on
  alfa/beta Ü> d/q : Subsystem  SimViewingDevice=off
  "angle " : Fcn  Expr=atan2(u[2],u[1])
  "mod " : Fcn  Expr=sqrt(u[1]^2+u[2]^2)
  mod : Outport  Port=1  InitialOutput=0
  angle : Outport  Port=2  InitialOutput=0
  emf : Outport  Port=3  InitialOutput=0
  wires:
  "angle "/1 -> angle/1, Gain/1
  rect/1 -> "angle "/1, "mod "/1, Derivative/1
  "mod "/1 -> mod/1
  Gain/1 -> alfa/beta Ü> d/q/2(angle)
  Derivative/1 -> alfa/beta Ü> d/q/1(vect)
  alfa/beta Ü> d/q/1(Out) -> emf/1

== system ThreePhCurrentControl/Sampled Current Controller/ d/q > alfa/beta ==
  vect : Inport  Port=1  PortDimensions=-1  SampleTime=-1  DataType=auto
  angle : Inport  Port=2  PortDimensions=-1  SampleTime=-1  DataType=auto
  Fcn : Fcn  Expr=u[1]*cos(u[3])-u[2]*sin(u[3])
  Fcn1 : Fcn  Expr=u[1]*sin(u[3])+u[2]*cos(u[3])
  Mux : Mux  Inputs=2
  Mux1 : Mux  Inputs=2
  Out : Outport  Port=1  InitialOutput=0
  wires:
  Mux1/1 -> Out/1
  Fcn1/1 -> Mux1/2
  Fcn/1 -> Mux1/1
  Mux/1 -> Fcn1/1, Fcn/1
  angle/1 -> Mux/2
  vect/1 -> Mux/1

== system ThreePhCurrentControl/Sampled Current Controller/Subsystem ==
  u : Inport  Orientation=left  Port=1  PortDimensions=-1  SampleTime=-1  DataType=auto
  Gammalt mätvärde2 : UnitDelay  Orientation=down  X0=0  SampleTime=Ts
  Gammalt mätvärde3 : UnitDelay  Orientation=left  X0=0  SampleTime=Ts
  Matsprediktor1 : Sum  Orientation=left  Inputs=+-  SaturateOnIntegerOverflow=on
  Proportional3 : Gain  Orientation=left  Gain=Ts/L  Multiplication=Element-wise(K.*u)  SaturateOnIntegerOverflow=on
  Proportional4 : Gain  Orientation=left  Gain=(1-Ts/(L/R))  Multiplication=Element-wise(K.*u)  SaturateOnIntegerOverflow=on
  Sum1 : Sum  Orientation=left  Inputs=++  SaturateOnIntegerOverflow=on
  di_smith : Outport  Orientation=left  Port=1
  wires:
  Proportional3/1 -> Sum1/1
  Proportional4/1 -> Sum1/2
  Sum1/1 -> Gammalt mätvärde2/1, Matsprediktor1/1
  u/1 -> Proportional3/1
  Matsprediktor1/1 -> Gammalt mätvärde3/1
  Gammalt mätvärde3/1 -> di_smith/1
  Gammalt mätvärde2/1 -> Proportional4/1, Matsprediktor1/2

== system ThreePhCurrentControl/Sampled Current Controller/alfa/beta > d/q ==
  vect : Inport  Port=1  PortDimensions=-1  SampleTime=-1  DataType=auto
  angle : Inport  Port=2  PortDimensions=-1  SampleTime=-1  DataType=auto
  Fcn : Fcn  Expr=u[1]*cos(u[3])-u[2]*sin(u[3])
  Fcn1 : Fcn  Expr=u[1]*sin(u[3])+u[2]*cos(u[3])
  Mux : Mux  Inputs=2
  Mux1 : Mux  Inputs=2
  Out : Outport  Port=1  InitialOutput=0
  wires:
  vect/1 -> Mux/1
  angle/1 -> Mux/2
  Mux/1 -> Fcn/1, Fcn1/1
  Fcn/1 -> Mux1/1
  Fcn1/1 -> Mux1/2
  Mux1/1 -> Out/1

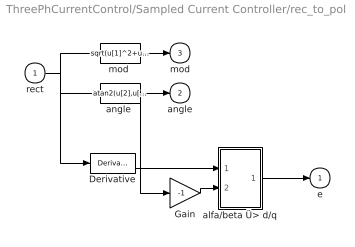
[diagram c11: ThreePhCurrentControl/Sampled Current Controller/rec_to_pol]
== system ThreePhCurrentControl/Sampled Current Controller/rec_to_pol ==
  rect : Inport  Port=1  PortDimensions=-1  SampleTime=-1  DataType=auto
  Derivative : Derivative
  Gain : Gain  Gain=-1  Multiplication=Element-wise(K.*u)  SaturateOnIntegerOverflow=on
  alfa/beta Ü> d/q : Subsystem  SimViewingDevice=off
  "angle " : Fcn  Expr=atan2(u[2],u[1])
  "mod " : Fcn  Expr=sqrt(u[1]^2+u[2]^2)
  e : Outport  Port=1  InitialOutput=0
  angle : Outport  Port=2  InitialOutput=0
  mod : Outport  Port=3  InitialOutput=0
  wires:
  "angle "/1 -> angle/1, Gain/1
  rect/1 -> "angle "/1, "mod "/1, Derivative/1
  "mod "/1 -> mod/1
  Gain/1 -> alfa/beta Ü> d/q/2(angle)
  Derivative/1 -> alfa/beta Ü> d/q/1(vect)
  alfa/beta Ü> d/q/1(Out) -> e/1

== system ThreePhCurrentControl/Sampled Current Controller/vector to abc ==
  vect : Inport  Port=1  PortDimensions=-1  SampleTime=-1  DataType=auto
  Ü> a : Fcn  Expr=sqrt(2/3)*u[1]
  Ü> b : Fcn  Expr=-sqrt(1/6)*u[1]+sqrt(1/2)*u[2]
  Ü> c : Fcn  Expr=-sqrt(1/6)*u[1]-sqrt(1/2)*u[2]
  a : Outport  Port=1  InitialOutput=0
  b : Outport  Port=2  InitialOutput=0
  c : Outport  Port=3  InitialOutput=0
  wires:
  vect/1 -> Ü> b/1, Ü> a/1, Ü> c/1
  Ü> b/1 -> b/1
  Ü> c/1 -> c/1
  Ü> a/1 -> a/1

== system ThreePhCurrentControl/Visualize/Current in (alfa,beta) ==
  xy : Inport  Port=1  PortDimensions=-1  SampleTime=-1  DataType=auto
  sfunxy : S-Function  FunctionName=sfunxy  Parameters=[xmin xmax ymin ymax], st  PortCounts=[]  SFunctionModules=''
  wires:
  xy/1 -> sfunxy/1

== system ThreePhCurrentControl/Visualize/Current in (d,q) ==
  xy : Inport  Port=1  PortDimensions=-1  SampleTime=-1  DataType=auto
  sfunxy : S-Function  FunctionName=sfunxy  Parameters=[xmin xmax ymin ymax], st  PortCounts=[]  SFunctionModules=''
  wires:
  xy/1 -> sfunxy/1

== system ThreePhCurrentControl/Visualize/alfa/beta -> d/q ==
  vect : Inport  Port=1  PortDimensions=-1  SampleTime=-1  DataType=auto
  angle : Inport  Port=2  PortDimensions=-1  SampleTime=-1  DataType=auto
  Fcn : Fcn  Expr=u[1]*cos(u[3])-u[2]*sin(u[3])
  Fcn1 : Fcn  Expr=u[1]*sin(u[3])+u[2]*cos(u[3])
  Mux : Mux  Inputs=2
  Mux1 : Mux  Inputs=2
  Out : Outport  Port=1  InitialOutput=0
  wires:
  vect/1 -> Mux/1
  angle/1 -> Mux/2
  Mux/1 -> Fcn/1, Fcn1/1
  Fcn/1 -> Mux1/1
  Fcn1/1 -> Mux1/2
  Mux1/1 -> Out/1

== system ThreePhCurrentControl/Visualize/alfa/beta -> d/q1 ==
  vect : Inport  Port=1  PortDimensions=-1  SampleTime=-1  DataType=auto
  angle : Inport  Port=2  PortDimensions=-1  SampleTime=-1  DataType=auto
  Fcn : Fcn  Expr=u[1]*cos(u[3])-u[2]*sin(u[3])
  Fcn1 : Fcn  Expr=u[1]*sin(u[3])+u[2]*cos(u[3])
  Mux : Mux  Inputs=2
  Mux1 : Mux  Inputs=2
  Out : Outport  Port=1  InitialOutput=0
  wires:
  Mux1/1 -> Out/1
  Fcn1/1 -> Mux1/2
  Fcn/1 -> Mux1/1
  Mux/1 -> Fcn1/1, Fcn/1
  angle/1 -> Mux/2
  vect/1 -> Mux/1

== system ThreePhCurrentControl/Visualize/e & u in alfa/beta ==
  xy : Inport  Port=1  PortDimensions=-1  SampleTime=-1  DataType=auto
  sfunxy : S-Function  FunctionName=sfunxy4  Parameters=[xmin xmax ymin ymax], st  PortCounts=[]  SFunctionModules=''
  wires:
  xy/1 -> sfunxy/1

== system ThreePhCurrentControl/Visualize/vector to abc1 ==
  vect : Inport  Port=1  PortDimensions=-1  SampleTime=-1  DataType=auto
  Ü> a : Fcn  Expr=sqrt(2/3)*u[1]
  Ü> b : Fcn  Expr=-sqrt(1/6)*u[1]+sqrt(1/2)*u[2]
  Ü> c : Fcn  Expr=-sqrt(1/6)*u[1]-sqrt(1/2)*u[2]
  a : Outport  Port=1  InitialOutput=0
  b : Outport  Port=2  InitialOutput=0
  c : Outport  Port=3  InitialOutput=0
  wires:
  Ü> a/1 -> a/1
  Ü> c/1 -> c/1
  Ü> b/1 -> b/1
  vect/1 -> Ü> c/1, Ü> a/1, Ü> b/1

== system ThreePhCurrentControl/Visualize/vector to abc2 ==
  vect : Inport  Port=1  PortDimensions=-1  SampleTime=-1  DataType=auto
  Ü> a : Fcn  Expr=sqrt(2/3)*u[1]
  Ü> b : Fcn  Expr=-sqrt(1/6)*u[1]+sqrt(1/2)*u[2]
  Ü> c : Fcn  Expr=-sqrt(1/6)*u[1]-sqrt(1/2)*u[2]
  a : Outport  Port=1  InitialOutput=0
  b : Outport  Port=2  InitialOutput=0
  c : Outport  Port=3  InitialOutput=0
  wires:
  vect/1 -> Ü> b/1, Ü> a/1, Ü> c/1
  Ü> b/1 -> b/1
  Ü> c/1 -> c/1
  Ü> a/1 -> a/1

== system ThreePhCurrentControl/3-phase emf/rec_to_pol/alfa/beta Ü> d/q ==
  vect : Inport  Port=1  PortDimensions=-1  SampleTime=-1  DataType=auto
  angle : Inport  Port=2  PortDimensions=-1  SampleTime=-1  DataType=auto
  Fcn : Fcn  Expr=u[1]*cos(u[3])-u[2]*sin(u[3])
  Fcn1 : Fcn  Expr=u[1]*sin(u[3])+u[2]*cos(u[3])
  Mux : Mux  Inputs=2
  Mux1 : Mux  Inputs=2
  Out : Outport  Port=1  InitialOutput=0
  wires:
  vect/1 -> Mux/1
  angle/1 -> Mux/2
  Mux/1 -> Fcn/1, Fcn1/1
  Fcn/1 -> Mux1/1
  Fcn1/1 -> Mux1/2
  Mux1/1 -> Out/1

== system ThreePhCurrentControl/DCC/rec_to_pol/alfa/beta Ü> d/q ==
  vect : Inport  Port=1  PortDimensions=-1  SampleTime=-1  DataType=auto
  angle : Inport  Port=2  PortDimensions=-1  SampleTime=-1  DataType=auto
  Fcn : Fcn  Expr=u[1]*cos(u[3])-u[2]*sin(u[3])
  Fcn1 : Fcn  Expr=u[1]*sin(u[3])+u[2]*cos(u[3])
  Mux : Mux  Inputs=2
  Mux1 : Mux  Inputs=2
  Out : Outport  Port=1  InitialOutput=0
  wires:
  vect/1 -> Mux/1
  angle/1 -> Mux/2
  Mux/1 -> Fcn/1, Fcn1/1
  Fcn/1 -> Mux1/1
  Fcn1/1 -> Mux1/2
  Mux1/1 -> Out/1

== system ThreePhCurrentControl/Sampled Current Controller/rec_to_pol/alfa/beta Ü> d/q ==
  vect : Inport  Port=1  PortDimensions=-1  SampleTime=-1  DataType=auto
  angle : Inport  Port=2  PortDimensions=-1  SampleTime=-1  DataType=auto
  Fcn : Fcn  Expr=u[1]*cos(u[3])-u[2]*sin(u[3])
  Fcn1 : Fcn  Expr=u[1]*sin(u[3])+u[2]*cos(u[3])
  Mux : Mux  Inputs=2
  Mux1 : Mux  Inputs=2
  Out : Outport  Port=1  InitialOutput=0
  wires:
  vect/1 -> Mux/1
  angle/1 -> Mux/2
  Mux/1 -> Fcn/1, Fcn1/1
  Fcn/1 -> Mux1/1
  Fcn1/1 -> Mux1/2
  Mux1/1 -> Out/1
